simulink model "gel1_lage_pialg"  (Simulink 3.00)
settings: Solver=ode45  SolverMode=SingleTasking  StartTime=0.0  StopTime=1.75  FixedStep=0.0001  RelTol=1e-3  AbsTol=1e-6
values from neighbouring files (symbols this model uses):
  bm = 4    [PI_Par.m]    (also in Red_Par.m)
  K_St = 1/FD_Stern    (= 2.27848101266)    [PI_Par.m]    (also in Red_Par.m = 1/FD_Stern)
  KL = omd*sqrt((1-TR^2*omd^2)+4*dR^2*TR^2*omd^2)    [PI_Par.m]    (also in Red_Par.m)
  KP = (1/K_St)*(2*d*T_St-T)/T    (= 23.3767988889)    [PI_Par.m]
  KVor = 1    [PI_Par.m]    (also in Red_Par.m)
  qA = 0    [PI_Par.m]    (also in Red_Par.m)
  T_St = M_Stern/FD_Stern    (= 2.82860759494)    [PI_Par.m]    (also in Red_Par.m = M_Stern/FD_Stern)
  TA = 0.001    [PI_Par.m]
  tb = vm/bm    (= 0.5)    [PI_Par.m]    (also in Red_Par.m)
  te = tv+tb    (= 1.2853981634)    [PI_Par.m]    (also in Red_Par.m)
  TN = T*(2*d-T/T_St)    (= 0.0693971006366)    [PI_Par.m]
  tv = se/vm    (= 0.785398163397)    [PI_Par.m]    (also in Red_Par.m)
  Vorz = 1    [PI_Par.m]    (also in Red_Par.m)
  z0 = (1/KM)*(rh)    (= 1.25)    [PI_Par.m]    (also in Red_Par.m = (1/KM)*(rh))

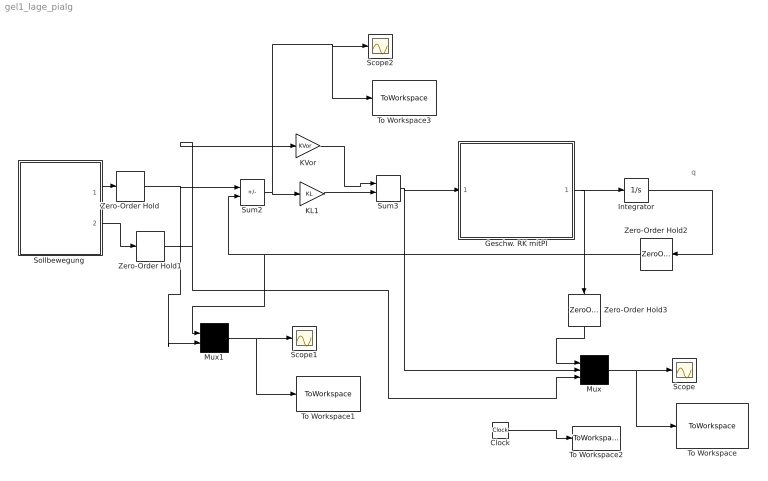
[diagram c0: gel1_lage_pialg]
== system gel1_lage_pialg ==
  note: q
  Clock : Clock
  Geschw. RK mitPI : Subsystem
  Integrator : Integrator  ExternalReset=none  InitialConditionSource=internal  InitialCondition=0  LimitOutput=off  UpperSaturationLimit=inf  LowerSaturationLimit=-inf  ShowSaturationPort=off  ShowStatePort=off  AbsoluteTolerance=auto
  KL1 : Gain  Gain=KL  SaturateOnIntegerOverflow=on
  KVor : Gain  Gain=KVor  SaturateOnIntegerOverflow=on
  Mux : Mux  Inputs=3
  Mux1 : Mux  Inputs=2
  Scope : Scope
  Scope1 : Scope
  Scope2 : Scope
  "Sollbewegung " : Subsystem
  Sum2 : Sum  Inputs=+-  SaturateOnIntegerOverflow=on
  Sum3 : Sum  Inputs=++  SaturateOnIntegerOverflow=on
  To Workspace : ToWorkspace  VariableName=Geschw_PI_M_Min  SampleTime=0.001  SaveFormat=Matrix
  To Workspace1 : ToWorkspace  VariableName=Lage_PI_M_Min  SampleTime=0.001  SaveFormat=Matrix
  To Workspace2 : ToWorkspace  VariableName=Zeit_Lage  SampleTime=0.001  SaveFormat=Matrix
  To Workspace3 : ToWorkspace  VariableName=e_PI_M_Min  SampleTime=0.001  SaveFormat=Matrix
  Zero-Order Hold : ZeroOrderHold  SampleTime=TA
  Zero-Order Hold1 : ZeroOrderHold  SampleTime=TA
  Zero-Order Hold2 : ZeroOrderHold  Orientation=left  SampleTime=TA
  Zero-Order Hold3 : ZeroOrderHold  Orientation=down  SampleTime=TA
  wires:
  Clock/1 -> To Workspace2/1
  KL1/1 -> Sum3/2
  KVor/1 -> Sum3/1
  Mux1/1 -> To Workspace1/1, Scope1/1
  Sum3/1 -> Geschw. RK mitPI/1(qps), Mux/2
  Sum2/1 -> KL1/1, Scope2/1, To Workspace3/1
  "Sollbewegung "/1(qS) -> Zero-Order Hold/1
  Zero-Order Hold/1 -> Sum2/1, Mux1/2
  "Sollbewegung "/2(qpss) -> Zero-Order Hold1/1
  Integrator/1 -> Zero-Order Hold2/1
  Zero-Order Hold2/1 -> Sum2/2, Mux1/1
  Mux/1 -> Scope/1, To Workspace/1
  Geschw. RK mitPI/1(v) -> Integrator/1, Zero-Order Hold3/1
  Zero-Order Hold3/1 -> Mux/1
  Zero-Order Hold1/1 -> KVor/1, Mux/3

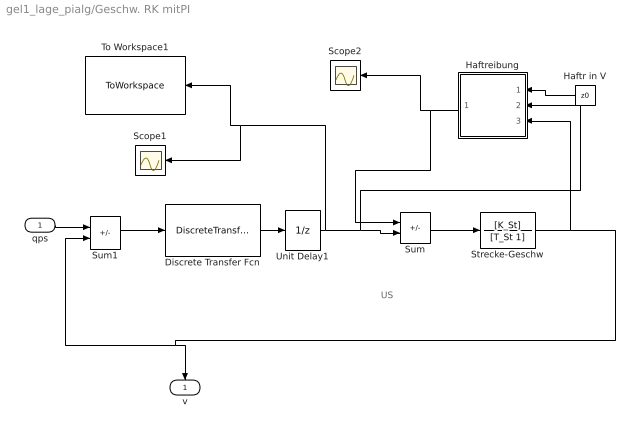
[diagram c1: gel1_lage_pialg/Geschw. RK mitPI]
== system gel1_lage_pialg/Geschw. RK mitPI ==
  note: US
  qps : Inport  Port=1  PortWidth=-1  SampleTime=-1  DataType=auto
  Discrete Transfer Fcn : DiscreteTransferFcn  Numerator=[KP -KP*(1-TA/TN)]  Denominator=[1 -1]  SampleTime=TA
  Haftr in V : Constant  Orientation=left  Value=z0
  Haftreibung : Subsystem  Orientation=left
  Scope1 : Scope
  Scope2 : Scope
  Strecke-Geschw : TransferFcn  Numerator=[K_St]  Denominator=[T_St 1]
  Sum : Sum  Inputs=-+  SaturateOnIntegerOverflow=on
  Sum1 : Sum  Inputs=+-  SaturateOnIntegerOverflow=on
  To Workspace1 : ToWorkspace  VariableName=Lage_PI_M_Min_US  SampleTime=0.001  SaveFormat=Matrix
  Unit Delay1 : UnitDelay  X0=0  SampleTime=TA
  v : Outport  Orientation=down  Port=1
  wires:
  qps/1 -> Sum1/1
  Sum/1 -> Strecke-Geschw/1
  Haftr in V/1 -> Haftreibung/1(z0)
  Sum1/1 -> Discrete Transfer Fcn/1
  Haftreibung/1(Out1) -> Scope2/1, Sum/1
  Discrete Transfer Fcn/1 -> Unit Delay1/1
  Unit Delay1/1 -> To Workspace1/1, Scope1/1, Sum/2, Haftreibung/2(US)
  Strecke-Geschw/1 -> Sum1/2, v/1, Haftreibung/3(qp)

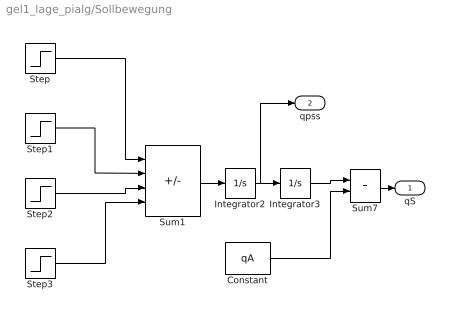
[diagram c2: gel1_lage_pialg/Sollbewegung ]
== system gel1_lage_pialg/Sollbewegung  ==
  Constant : Constant  Value=qA
  Integrator2 : Integrator  ExternalReset=none  InitialConditionSource=internal  InitialCondition=0  LimitOutput=off  UpperSaturationLimit=inf  LowerSaturationLimit=-inf  ShowSaturationPort=off  ShowStatePort=off  AbsoluteTolerance=auto
  Integrator3 : Integrator  ExternalReset=none  InitialConditionSource=internal  InitialCondition=0  LimitOutput=off  UpperSaturationLimit=inf  LowerSaturationLimit=-inf  ShowSaturationPort=off  ShowStatePort=off  AbsoluteTolerance=auto
  Step : Step  Time=0  Before=0  After=bm*Vorz  SampleTime=0.005
  Step1 : Step  Time=tb  Before=0  After=bm*Vorz  SampleTime=0.005
  Step2 : Step  Time=tv  Before=0  After=bm*Vorz  SampleTime=0.005
  Step3 : Step  Time=te  Before=0  After=bm*Vorz  SampleTime=0.005
  Sum1 : Sum  Inputs=+--+  SaturateOnIntegerOverflow=on
  Sum7 : Sum  Inputs=++  SaturateOnIntegerOverflow=on
  qS : Outport  Port=1  InitialOutput=0
  qpss : Outport  Port=2
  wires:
  Step/1 -> Sum1/1
  Step1/1 -> Sum1/2
  Step2/1 -> Sum1/3
  Step3/1 -> Sum1/4
  Sum1/1 -> Integrator2/1
  Integrator2/1 -> Integrator3/1, qpss/1
  Constant/1 -> Sum7/2
  Integrator3/1 -> Sum7/1
  Sum7/1 -> qS/1

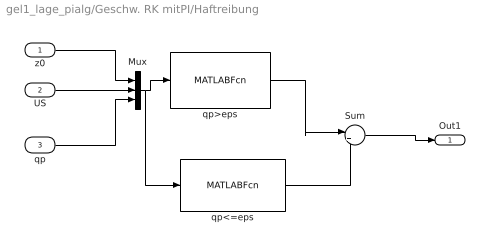
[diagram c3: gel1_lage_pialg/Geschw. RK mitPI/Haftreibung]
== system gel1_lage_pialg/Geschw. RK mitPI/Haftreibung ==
  z0 : Inport  Port=1  PortWidth=-1  SampleTime=-1  DataType=auto
  US : Inport  Port=2  PortWidth=-1  SampleTime=-1  DataType=auto
  qp : Inport  Port=3  PortWidth=-1  SampleTime=-1  DataType=auto
  Mux : Mux  Inputs=3
  Sum : Sum  Inputs=|++  SaturateOnIntegerOverflow=on
  qp<=eps : MATLABFcn  MATLABFcn=(abs(u(3)) < eps) *min(abs(u(2)),u(1))* sign(u(2))*sign(u(1))  OutputWidth=1  OutputSignalType=auto
  qp>eps : MATLABFcn  MATLABFcn=(abs(u(3)) > eps) * sign(u(3))*u(1)  OutputWidth=1  OutputSignalType=auto
  Out1 : Outport  Port=1  InitialOutput=0
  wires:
  z0/1 -> Mux/1
  US/1 -> Mux/2
  qp/1 -> Mux/3
  Mux/1 -> qp>eps/1, qp<=eps/1
  Sum/1 -> Out1/1
  qp>eps/1 -> Sum/1
  qp<=eps/1 -> Sum/2
